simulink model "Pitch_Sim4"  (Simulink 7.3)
settings: Solver=ode45  StartTime=0.0  StopTime=200  RelTol=1e-3
InitFcn:
  | init
StartFcn:
  | init
StopFcn:
  | pl
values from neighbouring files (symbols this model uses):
  d2r = 1/r2d    (= 0.0174532925199)    [init.m]    (also in freq.m; frequ.m; init_lat.m; pl.m)
undefined symbols (not defined in the file or in its folder): Ac, Ap, Bc, Bp, Cc, Cp, Dc, Dp

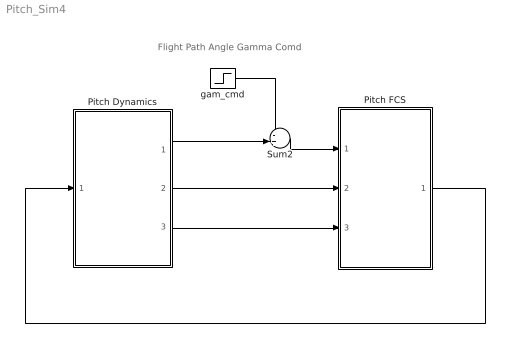
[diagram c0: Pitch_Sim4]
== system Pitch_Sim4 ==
  note: Flight Path Angle Gamma Comd
  Pitch Dynamics : Subsystem
  Pitch FCS : Subsystem
  Sum2 : Sum  Inputs=-+|  OutDataType=fixdt(1, 16)  OutScaling=2^0
  gam_cmd : Step  After=d2r  SampleTime=0
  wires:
  Pitch Dynamics/2(q) -> Pitch FCS/2(q)
  Pitch Dynamics/3(Nz) -> Pitch FCS/3(Nz)
  Pitch Dynamics/1(gamma) -> Sum2/2
  Sum2/1 -> Pitch FCS/1(gamerr)
  gam_cmd/1 -> Sum2/1
  Pitch FCS/1(d-elev) -> Pitch Dynamics/1(elev)

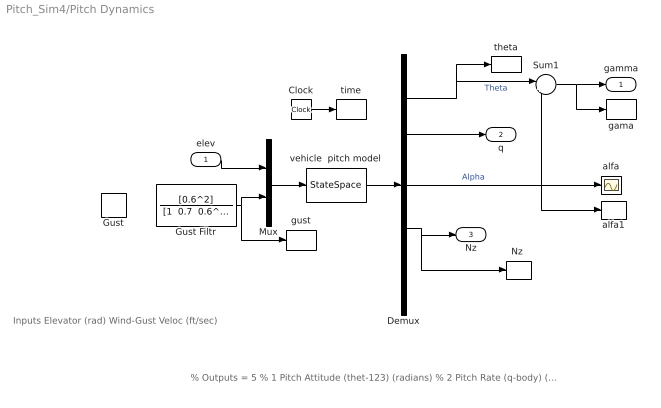
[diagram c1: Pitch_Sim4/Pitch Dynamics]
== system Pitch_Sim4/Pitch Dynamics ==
  note: % Outputs = 5 % 1 Pitch Attitude (thet-123) (radians) % 2 Pitch Rate (q-body) (rad/sec) % 3 Angle of attack, alfa, (radians) % 4 Accelerom # 2, (along Z), (ft/sec^2) Translat. Acceler % 5 Alpha Sensed at Vane # 1 (radian)
  note: Inputs Elevator (rad) Wind-Gust Veloc (ft/sec)
  elev : Inport
  Clock : Clock
  Demux : Demux  Outputs=5
  Gust : DiscretePulseGenerator  PulseType=Time based  Amplitude=30  Period=500  PulseWidth=2  PhaseDelay=0  SampleTime=1
  Gust Filtr : TransferFcn  Numerator=[0.6^2]  Denominator="[1  0.7  0.6^2]"
  Mux : Mux  Inputs=2
  "Nz " : ToWorkspace  VariableName=Nz  SampleTime=-1  SaveFormat=Array
  Sum1 : Sum  Inputs=|+-  OutDataType=fixdt(1, 16)  OutScaling=2^0
  alfa : Scope
  alfa1 : ToWorkspace  VariableName=alfa  SampleTime=-1  SaveFormat=Array
  gama : ToWorkspace  VariableName=gama  SampleTime=-1  SaveFormat=Array
  gust : ToWorkspace  VariableName=Vgst  SampleTime=-1  SaveFormat=Array
  theta : ToWorkspace  VariableName=theta  SampleTime=-1  SaveFormat=Array
  time : ToWorkspace  VariableName=time  SampleTime=-1  SaveFormat=Array
  vehicle  pitch model : StateSpace  A=Ap  B=Bp  C=Cp  D=Dp
  gamma : Outport
  q : Outport  Port=2
  Nz : Outport  Port=3
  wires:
  vehicle  pitch model/1 -> Demux/1
  Mux/1 -> vehicle  pitch model/1
  Demux/2 -> q/1
  elev/1 -> Mux/1
  Demux/3 -> Sum1/2, alfa/1, alfa1/1  "Alpha"
  Demux/4 -> Nz/1, "Nz "/1
  Sum1/1 -> gamma/1, gama/1
  Demux/1 -> Sum1/1, theta/1  "Theta"
  Gust Filtr/1 -> Mux/2, gust/1
  Clock/1 -> time/1

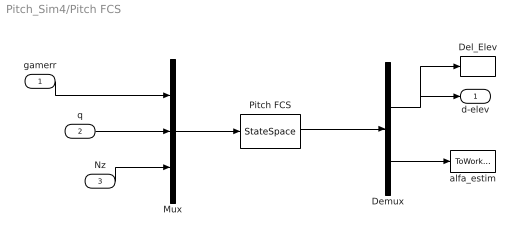
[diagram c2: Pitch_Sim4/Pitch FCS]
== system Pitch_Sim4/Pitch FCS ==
  gamerr : Inport
  q : Inport  Port=2
  Nz : Inport  Port=3
  Del_Elev : ToWorkspace  VariableName=delev  SampleTime=-1  SaveFormat=Array
  Demux : Demux  Outputs=2
  Mux : Mux  Inputs=3
  Pitch FCS : StateSpace  A=Ac  B=Bc  C=Cc  D=Dc
  alfa_estim : ToWorkspace  VariableName=alfa_est  SampleTime=-1  SaveFormat=Array
  d-elev : Outport
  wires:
  Nz/1 -> Mux/3
  Mux/1 -> Pitch FCS/1
  gamerr/1 -> Mux/1
  q/1 -> Mux/2
  Pitch FCS/1 -> Demux/1
  Demux/1 -> d-elev/1, Del_Elev/1
  Demux/2 -> alfa_estim/1
